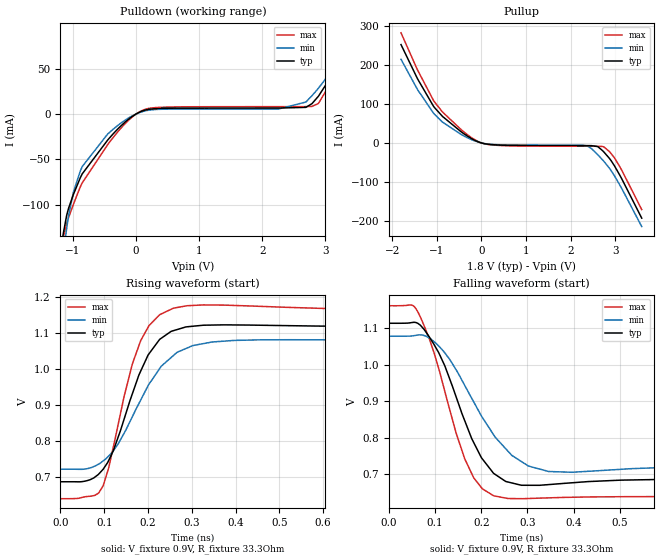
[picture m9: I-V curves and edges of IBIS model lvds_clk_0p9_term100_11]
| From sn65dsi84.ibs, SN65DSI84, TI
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|   Model
[Model]   lvds_clk_0p9_term100_11
Model_type   Output
Polarity   Non-Inverting
Vmeas = 0.9
Vref = 0.9
Cref = 1pF
Rref = 50
|   typ   min   max
C_comp   0.4797pF   0.3035pF   0.7186pF
[Voltage Range]   1.8   1.65   1.95
[Temperature Range]   27   125   -40
[Pullup Reference]   1.8   1.65   1.95
[Pulldown Reference]   -0   -0   -0
[Power Clamp Reference]   1.8   1.65   1.95
[GND Clamp Reference]   -0   -0   -0
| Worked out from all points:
|   slope of the pulldown table from 0 to 0.27 V, typ, clamps not added: 47.8 ohm
|   slope of the pullup table from 0 to 0.27 V, typ, clamps not added: 57.3 ohm
|   falling waveform, V_fixture 0.9V, R_fixture 33.3Ohm: 20-80 % time 80.2ps typ, 101ps min, 72.8ps max; typ from 1.11 V to 0.686 V
|   rising waveform, V_fixture 0.9V, R_fixture 33.3Ohm: 20-80 % time 76.3ps typ, 98.3ps min, 63.5ps max; typ from 0.686 V to 1.11 V
[Pulldown]
|   Voltage   I(typ)   I(min)   I(max)
-1.8V     -663.1mA   -698.1mA   -653.7mA
-1.152V   -130.3mA   -153.7mA   -135.1mA
-1.103V   -112.2mA   -126.9mA   -121mA
-995.4mV  -88.66mA   -86.15mA   -99.51mA
-855mV    -65.93mA   -57.85mA   -75.74mA
-450mV    -28.59mA   -21.99mA   -33.64mA
-93.6mV   -4.361mA   -3.333mA   -5.242mA
306mV     5.868mA    4.931mA    7.026mA
2.261V    6.534mA    5.501mA    8.066mA
2.693V    7.286mA    13.16mA    8.119mA
2.893V    19.56mA    28.36mA    11.59mA
3.595V    94.79mA    92.07mA    92.98mA
[Pullup]
|   Voltage   I(typ)   I(min)   I(max)
-1.8V     252.5mA    214.7mA    282.7mA
-1.427V   164.1mA    136.5mA    186.7mA
-1.055V   91.45mA    74.02mA    106mA
-860.4mV  67.05mA    52.52mA    78.31mA
-271.8mV  14.63mA    11.06mA    17.67mA
230.4mV   -4.388mA   -3.754mA   -5.088mA
2.374V    -7.009mA   -7.745mA   -8.528mA
2.612V    -9.74mA    -30.6mA    -8.676mA
2.752V    -24.09mA   -48.12mA   -10.65mA
2.914V    -46.63mA   -72.19mA   -28.09mA
3.152V    -93.27mA   -118.1mA   -71.16mA
3.595V    -193.2mA   -215mA     -171.2mA
[Ramp]
R_load = 33.3
|   typ   min   max
dV/dt_r   0.256987/7.62552e-11   0.214753/9.83071e-11   0.313206/6.34665e-11
dV/dt_f   0.25627/8.01968e-11   0.214196/1.01424e-10   0.313132/7.27688e-11
[Falling Waveform]
V_fixture = 0.9V
V_fixture_min = 0.9V
V_fixture_max = 0.9V
R_fixture = 33.3Ohm
C_fixture = 0F
|   Time   V(typ)   V(min)   V(max)
0s        1.113V     1.078V     1.161V
50ps      1.115V     1.079V     1.163V
63.2ps    1.112V     1.081V     1.143V
107.7ps   1.033V     1.051V     989.1mV
164.2ps   846.3mV    942.9mV    742.1mV
202.4ps   742mV      855.3mV    660.3mV
226.9ps   702.5mV    807.9mV    641.3mV
266.3ps   676.4mV    751.6mV    633.8mV
345.9ps   672mV      707.8mV    635.7mV
1ns       686mV      720.8mV    639.2mV
[Rising Waveform]
V_fixture = 0.9V
V_fixture_min = 0.9V
V_fixture_max = 0.9V
R_fixture = 33.3Ohm
C_fixture = 0F
|   Time   V(typ)   V(min)   V(max)
0s        686.1mV    720.9mV    639.2mV
78.53ps   699mV      729.4mV    648.4mV
97.65ps   721.2mV    744mV      675.3mV
120.9ps   772.7mV    772.6mV    783.5mV
164.2ps   930.2mV    866.7mV    1.013V
183.3ps   993.2mV    912.8mV    1.078V
226.6ps   1.081V     1V         1.149V
258ps     1.105V     1.036V     1.168V
396.2ps   1.121V     1.078V     1.175V
1ns       1.114V     1.079V     1.161V
